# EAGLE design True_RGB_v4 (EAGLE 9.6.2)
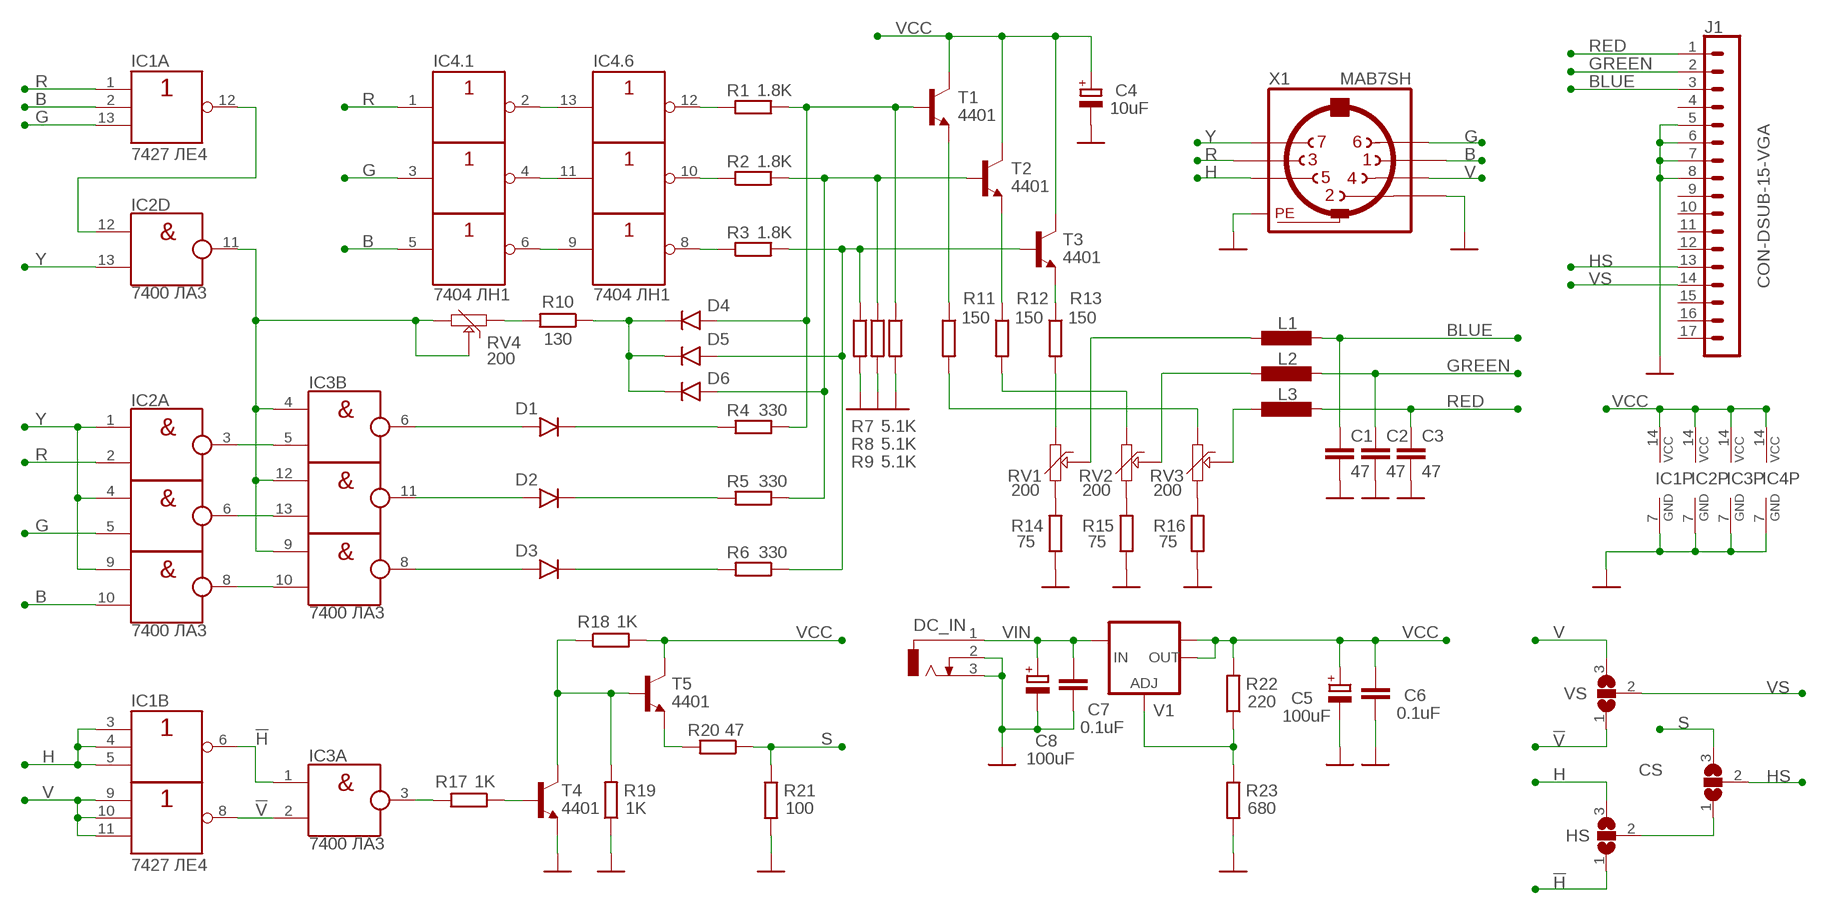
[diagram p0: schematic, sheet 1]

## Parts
C1  47  C-EU050-024X044  [C050-024X044]
C2  47  C-EU050-024X044  [C050-024X044]
C3  47  C-EU050-024X044  [C050-024X044]
C4  10uF  CPOL-EUE2.5-6  [E2,5-6]
C5  100uF  CPOL-EUE2.5-6  [E2,5-6]
C6  0.1uF  C-EU050-024X044  [C050-024X044]
C7  0.1uF  C-EU050-024X044  [C050-024X044]
C8  100uF  CPOL-EUE2.5-6  [E2,5-6]
CS  SJ2W  [SJ_2]
D1  1N4148AS  [D4148-2]
D2  1N4148AS  [D4148-2]
D3  1N4148AS  [D4148-2]
D4  1N4148AS  [D4148-2]
D5  1N4148AS  [D4148-2]
D6  1N4148AS  [D4148-2]
DC_IN  DCJ0202  [DCJ0202]
HS  SJ2W  [SJ_2]
IC1  7427 ЛЕ4  74HC27N  [DIL14]
IC2  7400 ЛА3  74HC00N  [DIL14]
IC3  7400 ЛА3  74HC00N  [DIL14]
IC4  7404 ЛН1  74HC04N  [DIL14]
J1  CON-DSUB-15-VGA  [181-015-212-171]
L1  0.56uH  L-EU0207/12  [0207/12]
L2  0.56uH  L-EU0207/12  [0207/12]
L3  0.56uH  L-EU0207/12  [0207/12]
R1  1.8K  R-EU_0207/2V  [0207/2V]
R2  1.8K  R-EU_0207/2V  [0207/2V]
R3  1.8K  R-EU_0207/2V  [0207/2V]
R4  330  R-EU_0207/2V  [0207/2V]
R5  330  R-EU_0207/2V  [0207/2V]
R6  330  R-EU_0207/2V  [0207/2V]
R7  5.1K  R-EU_0207/2V  [0207/2V]
R8  5.1K  R-EU_0207/2V  [0207/2V]
R9  5.1K  R-EU_0207/2V  [0207/2V]
R10  130  R-EU_0207/2V  [0207/2V]
R11  150  R-EU_0207/2V  [0207/2V]
R12  150  R-EU_0207/2V  [0207/2V]
R13  150  R-EU_0207/2V  [0207/2V]
R14  75  R-EU_0207/2V  [0207/2V]
R15  75  R-EU_0207/2V  [0207/2V]
R16  75  R-EU_0207/2V  [0207/2V]
R17  1K  R-EU_0207/2V  [0207/2V]
R18  1K  R-EU_0207/2V  [0207/2V]
R19  1K  R-EU_0207/2V  [0207/2V]
R20  47  R-EU_0207/2V  [0207/2V]
R21  100  R-EU_0207/2V  [0207/2V]
R22  220  R-EU_0207/2V  [0207/2V]
R23  680  R-EU_0207/2V  [0207/2V]
RV1  200  TRIM-6MM  [6MM]
RV2  200  TRIM-6MM  [6MM]
RV3  200  TRIM-6MM  [6MM]
RV4  200  TRIM-6MM  [6MM]
T1  4401  2N4401-NPN-TO92-EBC  [TO92-EBC]
T2  4401  2N4401-NPN-TO92-EBC  [TO92-EBC]
T3  4401  2N4401-NPN-TO92-EBC  [TO92-EBC]
T4  4401  2N4401-NPN-TO92-EBC  [TO92-EBC]
T5  4401  2N4401-NPN-TO92-EBC  [TO92-EBC]
V1  LM1117IMPX-ADJ  [SOT223]
VS  SJ2W  [SJ_2]
X1  MAB7SH  [MAB7SH]

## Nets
!H: HS.1 IC1.6(B:O) IC3.1(A:I0)
!V: IC1.8(C:O) IC3.2(A:I1) VS.1
B: IC1.2(A:I1) IC2.10(C:I1) IC4.5(.3:I) X1.1
BLUE: C1.1 J1.3 L1.1
G: IC1.13(A:I2) IC2.5(B:I1) IC4.3(.2:I) X1.6
GND: C1.2 C2.2 C3.2 C4.- C5.- C6.2 C7.2 C8.- DC_IN.2 DC_IN.3 IC1.7(P:GND) IC2.7(P:GND) IC3.7(P:GND) IC4.7(P:GND) J1.5 J1.6 J1.7 J1.8 R7.2 R8.2 R9.2 R14.1 R15.1 R16.1 R19.1 R21.2 R23.2 T4.E X1.2 X1.PE X1.PE@(PE)
GREEN: C2.1 J1.2 L2.1
H: HS.3 IC1.3(B:I0) IC1.4(B:I1) IC1.5(B:I2) X1.5
HS: CS.2 J1.13
N$1: D3.C R6.2
N$2: D2.C R5.2
N$3: D1.C R4.2
N$4: L1.2 RV1.S
N$5: IC1.12(A:O) IC2.12(D:I0)
N$6: CS.1 HS.2
N$7: L2.2 RV2.S
N$8: D5.A R3.2 R6.1 R7.1 T3.B
N$9: D6.A R2.2 R5.1 R8.1 T2.B
N$10: D4.A R1.2 R4.1 R9.1 T1.B
N$11: L3.2 RV3.S
N$12: R14.2 RV1.A
N$13: R15.2 RV2.A
N$14: R16.2 RV3.A
N$15: R11.1 T1.E
N$16: R12.2 RV2.E
N$17: R11.2 RV3.E
N$18: R12.1 T2.E
N$19: IC2.3(A:O) IC3.5(B:I1)
N$20: IC2.6(B:O) IC3.13(D:I1)
N$21: IC2.8(C:O) IC3.10(C:I1)
N$22: D1.A IC3.6(B:O)
N$23: D2.A IC3.11(D:O)
N$24: D3.A IC3.8(C:O)
N$25: IC4.2(.1:O) IC4.13(.6:I)
N$26: IC4.4(.2:O) IC4.11(.5:I)
N$27: IC4.6(.3:O) IC4.9(.4:I)
N$28: IC4.12(.6:O) R1.1
N$29: IC4.10(.5:O) R2.1
N$30: IC4.8(.4:O) R3.1
N$31: IC3.3(A:O) R17.2
N$32: R22.1 R23.1 V1.1(ADJ)
N$34: R17.1 T4.B
N$36: D4.C D5.C D6.C R10.1
N$37: R10.2 RV4.E
N$38: IC2.11(D:O) IC3.4(B:I0) IC3.9(C:I0) IC3.12(D:I0) RV4.A RV4.S
N$39: R13.1 T3.E
N$40: R13.2 RV1.E
N$176: R20.2 T5.E
N$177: R18.1 R19.2 T4.C T5.B
R: IC1.1(A:I0) IC2.2(A:I1) IC4.1(.1:I) X1.3
RED: C3.1 J1.1 L3.1
S: CS.3 R20.1 R21.1
V: IC1.9(C:I0) IC1.10(C:I1) IC1.11(C:I2) VS.3 X1.4
VCC: C4.+ C5.+ C6.1 IC1.14(P:VCC) IC2.14(P:VCC) IC3.14(P:VCC) IC4.14(P:VCC) R18.2 R22.2 T1.C T2.C T3.C T5.C V1.2(OUT) V1.TAB(OUT1)
VIN: C7.1 C8.+ DC_IN.1 V1.3(IN)
VS: J1.14 VS.2
Y: IC2.1(A:I0) IC2.4(B:I0) IC2.9(C:I0) IC2.13(D:I1) X1.7
Unconnected: J1.4 J1.9 J1.10 J1.11 J1.12 J1.15 J1.16 J1.17

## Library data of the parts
C1-C3 C6 C7 = rcl:C-EU: CAPACITOR, European symbol; SPICEPREFIX: C
C4 C5 C8 = rcl:CPOL-EU: POLARIZED CAPACITOR, European symbol; SPICEPREFIX: C
CS HS VS = jumper:SJ2W: SMD solder JUMPER
D1-D6 = 27C322:1N4148
DC_IN = power_jack:DCJ0202: DC POWER JACK Source: DCJ0202.pdf; OC_FARNELL: unknown; OC_NEWARK: unknown
IC1 = 74xx-eu:74*27: Triple 3-input NOR gate
IC2 IC3 = 74xx-eu:74*00: Quad 2-input NAND gate
IC4 = 74xx-eu:74*04: Hex INVERTER
J1 = m-pad-2.1:CON-DSUB-15-VGA: NORCOMP's High Density 90° PC Mount D-Sub Connector 181 Series: SPECIFICATIONS: Contact Rating: 5 Amps Dielectric Strength: 1000V AC RMS Insulation Resistance: 1000 meg ohms Contact Material: Phosphor Bronze Contact Finish: Gold flash over Nickel Operating Temperature: -55°C to 150°C Shell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
L1-L3 = rcl:L-EU: INDUCTOR, European symbol; SPICEPREFIX: L
R1-R23 = rcl:R-EU_: RESISTOR, European symbol; SPICEPREFIX: R
RV1-RV4 = 27C322:TRIM-6MM
T1-T5 = transistor-neu-to92:*-NPN-: NPN Transistror
V1 = lm1117:LM1117IMPX-ADJ
X1 = con-hirschmann:MAB7SH: Female CONNECTOR 7 pins with shield, horizontal (DIN 45329); OC_FARNELL: unknown; OC_NEWARK: unknown

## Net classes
1 power: width 0.66 mm, clearance 0.254 mm

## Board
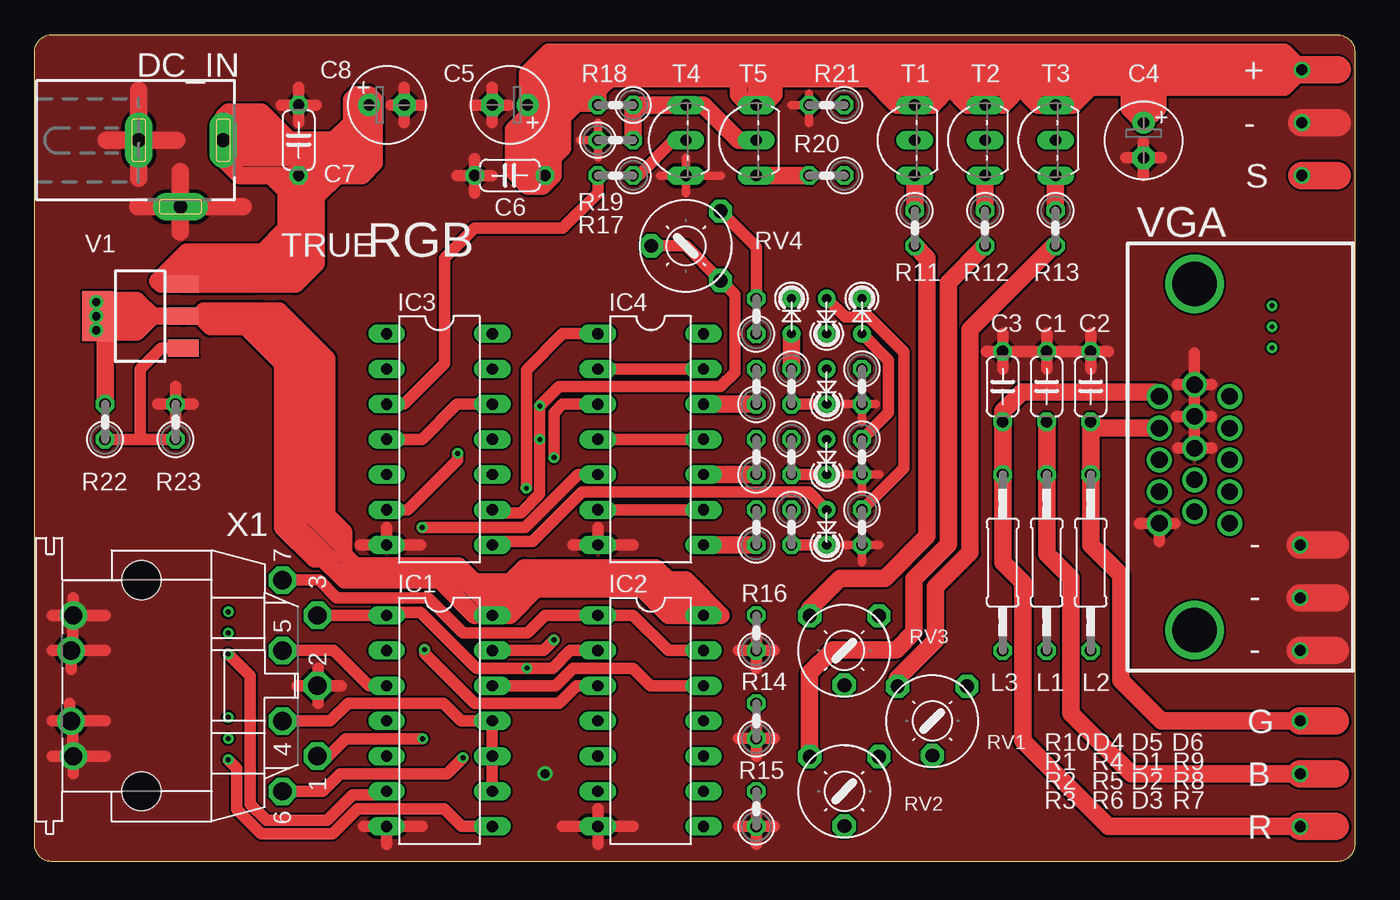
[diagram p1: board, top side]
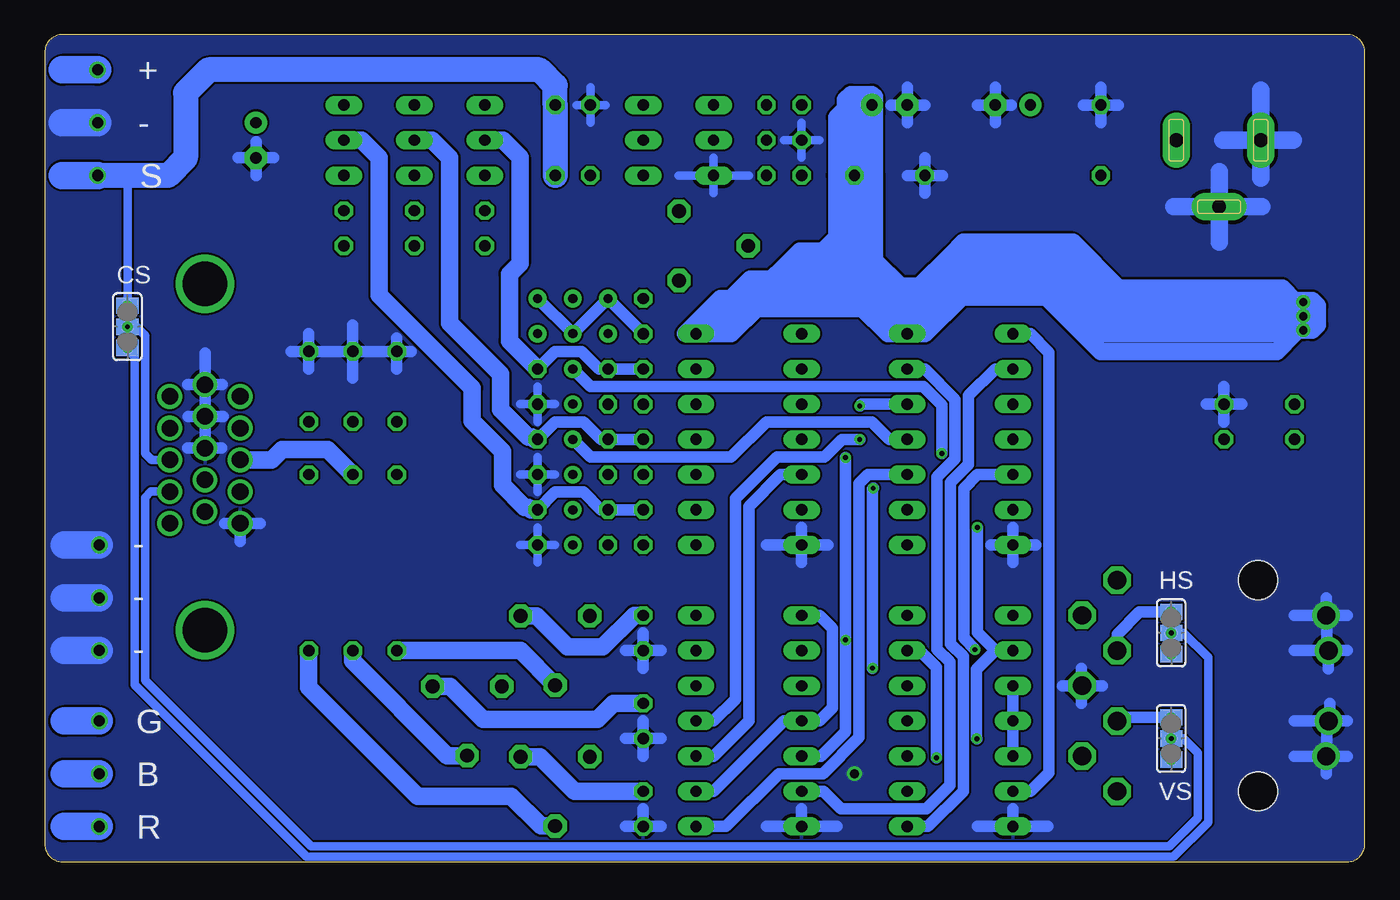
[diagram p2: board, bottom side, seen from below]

Size 95.25 x 59.69 mm. Coordinates in mm from the lower left corner, seen from the top.
Outline: 1.27,59.69 93.98,59.69 arc-90 95.25,58.42 95.25,1.27 arc-90 93.98,0 1.27,0 arc-90 0,1.27 0,58.42 arc-90 1.27,59.69
Copper layers (1*16): Top 0.035mm / dielectric 1.5mm / Bottom 0.035mm
Design rules "default *": minimum track width 6mil, minimum drill 0.35mm, track to track 6mil, track to pad 6mil, pad to pad 6mil, via to via 6mil, smd to smd 6mil, copper to edge 2mil, drill to drill 6mil, minimum pad ring 10mil, minimum via ring 8mil, stop-mask expansion 4mil, vias tented up to drill 20mil, thermal gap 10mil

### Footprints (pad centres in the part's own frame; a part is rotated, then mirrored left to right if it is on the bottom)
C050-024X044 = drill 0.813 octagon: 1 -2.54,0; 2 2.54,0
E2,5-6 = drill 0.813 pad 1.6: + -1.27,0 | drill 0.813 pad 1.6 octagon: - 1.27,0
SJ_2 = smd 1.168 x 1.6: 1 -1.524,0; 2 0,0; 3 1.524,0
D4148-2 = drill 0.65 pad 1.27: A 1.27,0; C -1.27,0
DCJ0202 = drill 1 pad 2 long: 1 0,3.1; 2 4.8,0; 3 0,-3
DIL14 = drill 0.813 long: 1 -7.62,-3.81; 2 -5.08,-3.81; 3 -2.54,-3.81; 4 0,-3.81; 5 2.54,-3.81; 6 5.08,-3.81; 7 7.62,-3.81; 8 7.62,3.81; 9 5.08,3.81; 10 2.54,3.81; 11 0,3.81; 12 -2.54,3.81; 13 -5.08,3.81; 14 -7.62,3.81
181-015-212-171 = drill 1.194: 1 4.371,2.541; 2 2.08,2.541; 3 -0.211,2.541; 4 -2.502,2.541; 5 -4.793,2.541; 6 5.217,0; 7 2.926,0; 8 0.635,0; 9 -1.656,0; 10 -3.947,0; 11 4.371,-2.541; 12 2.08,-2.541; 13 -0.211,-2.541; 14 -2.502,-2.541; 15 -4.793,-2.541 | drill 3.2: 16 -12.502,0; 17 12.502,0
0207/12 = drill 0.813 octagon: 1 -6.35,0; 2 6.35,0
0207/2V = drill 0.813 octagon: 1 -1.27,0; 2 1.27,0
6MM = drill 1 pad 1.676 octagon: A -2.5,-2.5; E 2.5,-2.5; S 0,2.5
TO92-EBC = drill 0.813 long: B 0,-1.27; C 2.54,-1.27; E -2.54,-1.27
SOT223 = smd 1.219 x 2.235: 1 -2.311,-3.099; 2 0,-3.099; 3 2.311,-3.099 | smd 3.6 x 2.2: TAB 0,3.099
MAB7SH = drill 1.321 octagon: 1 5.08,12.7; 2 0,12.7; 3 -5.08,12.7; 4 2.54,10.16; 5 -2.54,10.16; 6 7.62,10.16; 7 -7.62,10.16 | drill 1.321: PE -2.54,-5.08; PE@ 2.54,-5.08 | hole 2.794: 7.62,0; -7.62,0

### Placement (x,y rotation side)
C1  73.03,34.29 90 top
C2  76.2,34.29 90 top
C3  69.85,34.29 90 top
C4  80.01,52.07 270 top
C5  34.29,54.61 180 top
C6  34.29,49.53 180 top
C7  19.05,52.07 90 top
C8  25.4,54.61 0 top
CS  89.28,38.61 90 bottom
D1  57.15,34.29 90 top
D2  57.15,29.21 90 top
D3  57.15,24.13 90 top
D4  54.61,39.37 270 top
D5  57.15,39.37 90 top
D6  59.69,39.37 270 top
DC_IN  10.52,52.07 270 top
HS  13.97,16.51 90 bottom
IC1  29.21,10.16 270 top
IC2  44.45,10.16 270 top
IC3  29.21,30.48 270 top
IC4  44.45,30.48 270 top
J1  83.69,29.21 90 top
L1  73.03,21.59 270 top
L2  76.2,21.59 270 top
L3  69.85,21.59 270 top
R1  52.07,34.29 90 top
R2  52.07,29.21 90 top
R3  52.07,24.13 90 top
R4  54.61,34.29 270 top
R5  54.61,29.21 270 top
R6  54.61,24.13 270 top
R7  59.69,24.13 270 top
R8  59.69,29.21 270 top
R9  59.69,34.29 270 top
R10  52.07,39.37 90 top
R11  63.5,45.72 270 top
R12  68.58,45.72 270 top
R13  73.66,45.72 270 top
R14  52.07,10.16 90 top
R15  52.07,3.81 90 top
R16  52.07,16.51 90 top
R17  41.91,49.53 180 top
R18  41.91,54.61 180 top
R19  41.91,52.07 0 top
R20  57.15,49.53 180 top
R21  57.15,54.61 180 top
R22  5.08,31.75 90 top
R23  10.16,31.75 90 top
RV1  64.77,10.16 180 top
RV2  58.42,5.08 180 top
RV3  58.42,15.24 180 top
RV4  46.99,44.45 90 top
T1  62.23,52.07 90 top
T2  67.31,52.07 90 top
T3  72.39,52.07 90 top
T4  45.72,52.07 90 top
T5  50.8,52.07 90 top
V1  7.62,39.37 90 top
VS  13.97,8.89 90 bottom
X1  7.71,12.7 270 top

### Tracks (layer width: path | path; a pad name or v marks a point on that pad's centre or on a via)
!H  (via drill 0.35)
  Top 0.813: IC1.6 25.15,4.83 22.95,4.83 21.11,2.98 16.73,2.98 15.56,4.16 15.56,13.4 HS.1
  Bottom 0.813: IC3.1 24.13,38.1 22.78,36.75 22.78,6.43 24.13,5.08 IC1.6
  other vias: 13.97,14.99
!V  (via drill 0.35)
  Top 0.813: IC1.8 30.81,2.54 29.54,3.81 23.3,3.81 21.51,2.02 16.33,2.02 14.58,3.77 14.58,6.76 VS.1
  Bottom 0.813: IC1.8 31.52,2.54 28.98,5.08 28.98,14.82 29.9,15.73 29.9,27.37 28.6,28.66 28.6,33.63 26.67,35.56 IC3.2
  other vias: 13.97,7.37
B  (via drill 0.35)
  Top 0.813: IC4.5 39.21,27.94 35.4,24.13 v27.97,24.13 | v28,8.88 22.43,8.88 21.17,7.62 X1.1
  Bottom 0.813: IC2.10 46.99,7.62 44.45,10.16 44.45,25.65 42.16,27.94 IC4.5 | IC1.2 26.64,15.24 | v27.97,24.13 v27.96,24.13 27.96,16.56 26.64,15.24 | 26.64,15.24 28.01,13.87 28.01,8.89 v28,8.88
BLUE  (via drill 0.8)
  Top 1.27: C1.1 L1.1 73.03,22.23 74.75,20.5 74.75,10.72 79.12,6.35 v91.31,6.35
  Top 2: v91.31,6.35 93.85,6.35
  Bottom 1.27: L1.1 74.85,29.76 78.1,29.76 78.87,29 J1.3
  Bottom 2: v91.31,6.35 93.85,6.35
G  (via drill 0.35)
  Top 0.813: IC4.3 38.09,33.02 37.47,32.4 v37.47,29.16 | X1.6 20.78,5.08 22.05,6.35 29.76,6.35 v30.91,7.5 | v37.47,16 36.7,15.24 IC1.13
  Bottom 0.813: IC2.5 39.23,7.62 37.47,9.38 v37.47,16 v37.47,29.16 | v30.91,7.5 30.91,14.02 32.13,15.24 IC1.13
GND  (via drill 0.65, 0.8, 1.3 pad 2)
  Top 0.61: R9.2 60.71,33.02 | R9.2 59.69,34.29 | R9.2 58.42,33.02 | R9.2 59.69,31.75 | R8.2 60.96,27.94 | R8.2 59.69,29.21 | R8.2 58.42,27.94 | R8.2 59.69,26.67 | R7.2 60.96,22.86 | R7.2 59.69,24.13 | R7.2 58.42,22.86 | R7.2 59.69,21.59 | T4.E 46.99,48.26 | T4.E 45.11,49.53 | T4.E 49.53,49.53 | T4.E 46.99,50.8 | R21.2 55.88,53.29 | R21.2 54.61,54.61 | R21.2 57.15,54.61 | R19.1 39.37,52.07 | R19.1 40.64,53.34 | R19.1 40.64,50.8 | R19.1 41.91,52.07 | R21.2 55.88,55.42
  Top 0.813: C5.- 33.02,55.88 | C5.- 31.75,54.61 | C5.- 34.2,54.61 | C5.- 33.02,53.34 | C6.2 31.75,50.75 | C6.2 30.48,49.53 | C6.2 33.02,49.53 | C6.2 31.75,48.26 | IC4.7 38.86,22.86 | IC4.7 40.64,24.13 | IC4.7 43.18,22.86 | C4.- 80.01,51.98 | C4.- 80.01,49.53 | C4.- 81.28,50.8 | C4.- 78.74,50.8 | C3.2 69.85,38.1 | C3.2 C1.2 | C3.2 69.85,35.56 | C1.2 73.03,35.56 | C1.2 73.03,38.1 | C2.2 C1.2 | C2.2 77.47,36.83 | C2.2 76.2,38.1 | C2.2 76.2,35.56 | C3.2 68.68,36.83 | R16.1 50.8,15.24 | R16.1 52.07,16.51 | R16.1 53.34,15.24 | R16.1 52.07,13.97 | R14.1 52.07,7.62 | R14.1 52.07,10.16 | R14.1 50.8,8.89 | R14.1 53.34,8.89 | R15.1 52.07,3.81 | R15.1 52.07,1.27 | R15.1 53.34,2.54 | R15.1 50.8,2.54 | IC2.7 38.1,2.54 | IC2.7 43.18,2.54 | IC2.7 40.64,1.27 | IC2.7 40.64,3.81 | IC1.7 27.94,2.54 | IC1.7 25.4,1.27 | IC3.7 27.84,22.86 | IC3.7 25.4,24.13 | X1.2 18.92,12.7 | 20.45,13.97 20.45,12.74 X1.2 | X1.2 20.45,12.66 20.45,11.43 | X1.2 22.1,12.7 | v2.79,7.62 1.27,7.62 | v2.79,7.62 5.08,7.62 | X1.PE@ 5.08,10.16 | X1.PE@ 1.27,10.16 | X1.PE@ 2.54,10.25 2.54,11.43 | X1.PE@ 2.76,10.03 2.76,7.66 v2.79,7.62 | v2.79,7.62 2.79,6.35 | X1.PE 2.63,13.88 | X1.PE 2.76,15.37 2.76,17.74 v2.79,17.78 | X1.PE 1.27,15.24 | X1.PE 5.08,15.24 | v2.79,17.78 5.08,17.78 | v2.79,17.78 1.27,17.78 | v2.79,17.78 2.79,19.05 | R23.2 10.16,34.29 | R23.2 10.16,31.75 | R23.2 11.43,33.02 | R23.2 8.89,33.02 | C7.2 19.05,55.88 | C7.2 19.05,53.34 | C7.2 20.32,54.61 | C7.2 17.78,54.61 | C8.- 26.67,55.88 | C8.- 27.94,54.61 | C8.- 26.67,53.34 | C8.- 25.7,54.61 | J1.6 J1.7 | J1.7 J1.8 | J1.6 83.69,36.7 | J1.6 84.95,34.43 | J1.6 82.43,34.43 | J1.8 82.49,29.84 | J1.8 84.92,29.84 | J1.7 82.36,32.14 | J1.7 84.9,32.14 | J1.5 81.15,23.11 | J1.5 79.72,24.42 | J1.5 82.26,24.42 | IC1.7 23.75,2.54 | IC3.7 23.5,22.86
  Top 1.27: DC_IN.3 7.52,55.67 | DC_IN.3 7.52,49.32 | DC_IN.3 10.26,52.07 | DC_IN.3 5.18,52.07 | DC_IN.2 10.52,49.78 | DC_IN.2 10.52,45.45 | DC_IN.2 7.44,47.27 | DC_IN.2 15.06,47.27
  Top 2: v91.44,53.34 93.98,53.34 | v91.31,15.24 93.85,15.24 | v91.31,19.05 93.85,19.05 | v91.31,22.86 93.85,22.86
  Bottom 0.61: R19.1 40.64,53.34 | R19.1 39.37,52.07 | R19.1 41.91,52.07 | R19.1 40.64,50.8 | T4.E 44.45,49.53 | T4.E 46.99,50.8 | T4.E 46.99,48.26 | T4.E 49.53,49.53 | R21.2 56.9,54.61 | R21.2 55.88,53.34 | R21.2 54.8,54.61 | R21.2 55.88,55.88 | R8.2 59.69,29.21 | R8.2 58.42,27.94 | R8.2 60.96,27.94 | R8.2 59.69,26.67 | R7.2 59.69,21.59 | R7.2 60.96,22.86 | R7.2 58.42,22.86 | R7.2 59.69,24.13 | R9.2 59.69,34.29 | R9.2 60.96,33.02 | R9.2 58.42,33.02 | R9.2 59.69,31.75
  Bottom 0.813: C6.2 30.48,49.53 | C6.2 33.02,49.53 | C6.2 31.75,50.8 | C5.- 33.02,55.88 | C5.- 34.2,54.61 | C5.- 31.75,54.61 | C5.- 33.02,53.34 | C4.- 78.74,50.8 | C4.- 80.01,49.53 | C4.- 81.28,50.8 | C4.- 80.01,51.98 | C3.2 68.83,36.83 | C3.2 C1.2 | C1.2 C2.2 | C2.2 77.47,36.83 | C2.2 76.2,38.1 | C2.2 76.2,35.56 | C1.2 73.03,38.73 | C1.2 73.03,34.92 | C3.2 69.85,37.8 | C3.2 69.85,35.56 | R16.1 52.07,13.97 | R16.1 50.8,15.24 | R16.1 53.34,15.24 | R16.1 52.07,16.51 | R14.1 52.07,10.16 | R14.1 53.34,8.89 | R14.1 50.8,8.89 | R14.1 52.07,7.62 | R15.1 50.8,2.54 | R15.1 52.07,3.81 | R15.1 53.34,2.54 | v2.79,7.62 5.08,7.62 | v2.79,7.62 1.27,7.62 | v2.79,7.62 2.79,6.35 | v2.79,7.62 2.76,7.66 2.76,10.03 X1.PE@ | X1.PE@ 2.54,10.25 2.54,11.43 | X1.PE 2.63,13.93 | X1.PE 2.76,15.37 2.76,17.74 v2.79,17.78 | v2.79,17.78 5.08,17.78 | v2.79,17.78 1.27,17.78 | v2.79,17.78 2.79,19.05 | X1.PE 5.08,15.24 | X1.PE 1.27,15.24 | X1.PE@ 5.08,10.16 | X1.PE@ 1.27,10.16 | X1.2 18.92,12.7 | 20.45,13.97 20.45,12.74 X1.2 | X1.2 20.45,12.66 20.45,11.43 | X1.2 21.82,12.7 | R23.2 11.43,33.02 | R23.2 8.89,33.02 | R23.2 10.16,34.29 | R23.2 10.16,31.75 | C7.2 19.05,55.88 | C7.2 19.05,53.34 | C7.2 20.32,54.61 | C7.2 17.78,54.61 | C8.- 26.67,55.88 | C8.- 26.67,53.34 | C8.- 25.49,54.61 | C8.- 27.94,54.61 | C6.2 31.75,48.26 | IC2.7 43.18,2.54 | IC2.7 40.64,3.81 | IC2.7 38.1,2.54 | IC1.7 27.94,2.54 | IC1.7 25.4,3.81 | IC1.7 22.86,2.54 | IC3.7 25.4,21.59 | IC3.7 25.4,24.13 | IC3.7 27,22.86 | IC3.7 23.75,22.86 | IC4.7 38.73,22.86 | IC4.7 40.64,24.13 | IC4.7 43.18,22.86 | IC4.7 40.64,21.59 | J1.6 J1.7 | J1.7 J1.8 | J1.6 83.69,36.7 | J1.6 84.95,34.43 | J1.6 82.43,34.43 | J1.8 82.49,29.84 | J1.8 84.92,29.84 | J1.7 82.36,32.14 | J1.7 84.9,32.14 | J1.5 81.15,23.11 | J1.5 79.72,24.42 | J1.5 82.26,24.42
  Bottom 1.27: DC_IN.3 7.52,55.67 | DC_IN.3 7.52,49.32 | DC_IN.2 10.52,49.78 | DC_IN.2 10.52,44.7 | DC_IN.2 13.79,47.27 | DC_IN.2 7.44,47.27 | DC_IN.3 5.18,52.07 | DC_IN.3 10.26,52.07
  Bottom 2: v91.44,53.34 93.98,53.34 | v91.31,15.24 93.85,15.24 | v91.31,19.05 93.85,19.05 | v91.31,22.86 93.85,22.86
  other vias: 36.83,6.35
  pour Bottom: -2.54,62.23 97.79,62.23 97.79,-2.54 -2.54,-2.54
  pour Top: -2.54,62.23 97.79,62.23 97.79,-2.54 -2.54,-2.54
GREEN  (via drill 0.8)
  Top 1.27: J1.2 76.71,31.29 76.2,31.8 C2.1 L2.1 76.2,22.86 78.36,20.7 78.36,13.08 81.28,10.16 v91.31,10.16
  Top 2: v91.31,10.16 93.85,10.16
  Bottom 2: v91.31,10.16 93.85,10.16
H  (via drill 0.35)
  Top 0.813: IC1.3 24.13,12.7 21.59,15.24 X1.5
  Bottom 0.813: IC1.3 IC1.4 IC1.5 | HS.3 16.26,18.03 17.87,16.42 X1.5
  other vias: 13.97,18.03
HS  (via drill 0.35)
  Bottom 0.61: J1.13 87.55,29 88.01,29.46 88.01,37.97 88.65,38.61 CS.2
  other vias: 89.28,38.61
N$1
  Top 0.813: R6.2 D3.C
N$2
  Top 0.813: R5.2 D2.C
N$3
  Top 0.813: R4.2 D1.C
N$4
  Bottom 1.27: L1.2 73.03,14.48 66.21,7.66 RV1.S
N$5
  Top 0.813: IC2.12 44.45,12.7 43.18,13.97 38.86,13.97 37.59,12.7 IC1.12
N$6  (via drill 0.35)
  Bottom 0.61: HS.2 13.08,16.51 11.3,14.73 11.3,2.86 13.81,0.36 76.36,0.36 88.77,12.77 88.77,36.45 89.28,36.96 CS.1
  other vias: 13.97,16.51 89.28,37.08
N$7
  Bottom 1.27: L2.2 76.2,12.57 68.37,4.74 61.59,4.74 59.44,2.58 RV2.S
N$8
  Top 0.813: D5.A 58.5,39.29 60.18,39.29 62.71,36.77 62.71,28.42 R7.1
  Bottom 0.813: R3.2 R6.1 55.12,25.4 56.39,26.67 58.42,26.67 R7.1
  Bottom 1.27: R7.1 60.18,25.4 60.35,25.58 60.63,25.58 62.23,27.18 62.23,29.61 64.41,31.8 64.41,34.19 71.12,40.89 71.12,50.8 72.39,52.07 T3.B
N$9
  Top 0.813: D6.A 61.62,36.17 61.62,32.41 R8.1
  Bottom 0.813: R2.2 R5.1 55.12,30.48 56.39,31.75 58.42,31.75 R8.1
  Bottom 1.27: R8.1 59.92,30.48 60.1,30.66 60.38,30.66 62.36,32.64 62.36,35.18 66.04,38.86 66.04,50.8 67.31,52.07 T2.B
N$10
  Top 1.27: D4.A R4.1
  Bottom 0.813: R1.2 R4.1 55.24,35.56 56.52,36.83 58.42,36.83 R9.1
  Bottom 1.27: R9.1 61.72,37.59 61.72,42.42 60.96,43.18 60.96,50.84 62.19,52.07 T1.B
N$11
  Bottom 1.27: RV3.S 60.92,15.24 L3.2
N$12
  Bottom 1.27: R14.2 54.23,11.43 55.37,10.29 63.63,10.29 66,12.66 RV1.A
N$13
  Bottom 1.27: RV2.A 59.52,7.58 57.02,5.08 R15.2
N$14
  Bottom 1.27: RV3.A 59.78,17.74 57.53,15.49 54.99,15.49 52.7,17.78 R16.2
N$15
  Top 1.27: T1.E R11.1
N$16
  Top 1.27: R12.2 65.94,41.81 65.94,22.91 63.44,20.4 63.44,16.57 62.17,15.3 57.59,15.3 55.92,13.63 RV2.E
N$17
  Top 1.27: R11.2 64.39,43.56 64.39,23.5 61.34,20.45 58.12,20.45 55.92,18.25 RV3.E
N$18
  Top 1.27: R12.1 T2.E
N$19  (via drill 0.35)
  Top 0.813: IC2.3 39.12,12.7 37.85,11.43 31.75,11.43 28.13,15.05 v28.13,15.31
  Bottom 0.813: IC3.5 27.94,27.94 28.93,26.95 28.93,16.14 28.13,15.33 v28.13,15.31
N$20
  Bottom 0.813: IC2.6 39.08,5.08 37.81,3.81 31.64,3.81 29.94,5.5 29.94,14.42 30.86,15.34 30.86,27.77 29.56,29.06 29.56,33.37 31.75,35.56 IC3.13
N$21
  Bottom 0.813: IC2.8 46.1,2.54 42.29,6.35 39.12,6.35 36.5,8.97 36.5,27.3 35.85,27.94 IC3.10
N$22  (via drill 0.35)
  Top 0.813: IC3.6 26.92,25.4 30.53,29 v30.53,29.46
  Bottom 0.813: D1.A 55.88,34.29 31.84,34.29 30.53,32.97 v30.53,29.46
N$23
  Bottom 0.813: D2.A 55.88,29.21 45.72,29.21 43.18,31.75 35.56,31.75 34.29,30.48 IC3.11
N$24
  Top 0.813: D3.A 55.88,26.67 39.5,26.67 35.93,23.1 33.26,23.1 IC3.8
N$25
  Top 0.813: IC4.2 IC4.13
N$26
  Top 0.813: IC4.4 IC4.11
N$27
  Top 0.813: IC4.6 IC4.9
N$28
  Top 1.27: IC4.12 R1.1
N$29
  Top 1.27: IC4.10 R2.1
N$30
  Top 1.27: IC4.8 R3.1
N$31
  Top 0.813: IC3.3 26.67,33.02 29.59,35.94 29.59,43.56 31.75,45.72 38.1,45.72 40.64,48.26 R17.2
N$32
  Top 0.813: V1.1 10.71,37.07 9.13,37.07 7.62,35.56 7.62,30.48 | R23.1 7.62,30.48 | 7.62,30.48 R22.1
N$34
  Top 0.813: R17.1 43.56,49.53 46.1,52.07 T4.B
N$36
  Bottom 0.813: R10.1 D4.C D5.C D6.C
N$37
  Top 0.813: R10.2 52.07,44.37 RV4.E
N$38  (via drill 0.35)
  Top 0.813: IC3.9 33.24,25.18 35.09,25.18 36.45,26.54 v36.45,30.48 v36.45,32.89 37.85,34.29 49.5,34.29 50.52,35.31 50.52,40.92 RV4.A 46.99,44.45 RV4.S | IC3.12 30.48,33.02 27.94,30.48 IC3.4
  Bottom 0.813: IC2.11 46.99,10.16 45.43,11.72 45.43,26.2 42.42,29.21 38.99,29.21 37.72,30.48 v36.45,30.48 | IC3.12 36.32,33.02 v36.45,32.89
N$39
  Top 1.27: T3.E R13.1
N$40
  Top 1.27: R13.2 73.53,44.45 67.49,38.41 67.49,22.32 64.99,19.82 64.99,15.96 62.27,13.25 RV1.E
  Bottom 1.27: R13.2 73.7,44.41
N$176
  Top 1.27: R20.2 T5.E
N$177
  Top 1.27: T5.B 50.8,52.07 48.26,54.61 T4.C R18.1 R19.2
R  (via drill 0.35)
  Top 0.813: IC2.2 38.64,15.24 37.37,13.97 v35.52,13.97 31.9,13.97 27.86,18.01 25.63,18.01 IC1.1 X1.3 | IC4.1 38.1,38.1 35.48,35.48 35.48,26.97 v35.47,26.96
  Bottom 0.813: v35.47,26.96 35.53,26.9 35.53,13.98 v35.52,13.97
RED  (via drill 0.8)
  Top 1.27: J1.1 80.82,33.91 71.25,33.91 69.85,32.51 C3.1 L3.1 69.85,21.59 71.3,20.14 71.3,8.71 77.47,2.54 v91.31,2.54
  Top 2: v91.31,2.54 93.85,2.54
  Bottom 2: v91.31,2.54 93.85,2.54
S  (via drill 0.35, 0.8)
  Top 2: 93.98,49.53 v91.44,49.53
  Bottom 0.61: v91.44,49.53 89.28,49.53 CS.3
  Bottom 1.8: v91.44,49.53 86.36,49.53 85.09,50.8 85.09,55.5 83.44,57.15 59.56,57.15 58.42,56.01 R21.1 R20.1
  Bottom 2: v91.44,49.53 93.98,49.53
  other vias: 89.28,40.13
V  (via drill 0.35)
  Top 0.813: IC1.9 IC1.10 IC1.11 30.77,10.16 29.5,11.43 22.61,11.43 21.34,10.16 X1.4
  Bottom 0.813: VS.3 17.61,10.41 X1.4
  other vias: 13.97,10.41
VCC  (via drill 0.6 pad 0.95, 0.8)
  Top 0.61: V1.TAB v4.44,39.37
  Top 0.813: 5.08,38.11 4.84,38.35 v4.44,38.35
  Top 1.27: 40.64,57.15 78.99,57.15 | 78.99,57.15 81.03,57.15 | 81.03,57.15 82.55,57.15 | 40.64,57.15 40.64,57.4 37.08,57.4 36.2,56.52 | 40.64,57.15 40.64,55.88 | 40.64,55.88 40.88,55.88 41.51,56.52 50.8,56.52 | 50.8,56.52 52.07,56.52 | 52.07,56.52 53.34,56.52 | 53.34,56.52 60.33,56.52 | 60.33,56.52 60.96,56.52 61.59,55.88 66.04,55.88 | T5.C 52.07,56.52 | T5.C 52.58,54.61 53.34,55.37 53.34,56.52 | T5.C 51.56,54.61 50.8,55.37 50.8,56.52 | 35.56,53.85 C5.+ 35.56,55.88 | 36.7,54.61 36.7,56.13 | 35.56,55.88 35.56,56.9 37.07,58.41 82.55,58.41 | 36.2,56.52 35.56,55.88 | 36.7,54.61 36.45,54.36 36.45,49.91 C6.1 | 36.7,54.61 37.4,55.31 | 40.64,55.88 37.4,55.88 37.4,55.31 | 36.2,56.52 38.1,56.52 | 38.1,56.52 40.01,56.52 40.64,57.15 | 35.56,53.85 34.54,52.83 34.54,49.78 35.56,48.77 36.64,48.77 37.4,49.53 | C6.1 36.7,49.66 | C6.1 37.4,49.53 | 37.4,49.53 37.4,50.8 | 37.4,50.8 37.4,55.31 | C6.1 35.56,49.53 35.56,53.85 | T2.C 67.31,54.61 66.04,55.88 | 71.12,55.88 69.85,54.61 | 71.12,55.88 72.39,54.61 T3.C 74.93,54.61 76.2,55.88 | 82.55,55.88 82.55,57.15 | 82.55,57.15 82.55,58.41 | 66.04,55.88 64.77,54.61 T1.C 62.23,54.61 60.33,56.52 | 66.04,55.88 71.12,55.88 | 71.12,55.88 76.2,55.88 | 82.55,58.41 90.18,58.41 v91.44,57.15 90.17,55.88 82.55,55.88 | 82.55,55.88 83.82,57.15 | 76.2,55.88 80.01,55.88 | 80.01,55.88 82.55,55.88 | 40.64,55.88 R18.2 40.51,54.74 39.12,54.74 38.1,53.72 | 38.1,56.52 38.1,53.72 | 38.1,53.72 38.1,51.5 37.4,50.8 | C4.+ 80.01,55.88 | C4.+ 78.99,54.36 78.99,57.15 | C4.+ 81.03,54.36 81.03,57.15 | 8.51,39.37 V1.2 11.94,39.37 | 8.51,39.37 V1.TAB | V1.TAB 5.66,40.51 7.37,40.51 8.51,39.37 | V1.TAB 4.52,38.66 4.95,38.23 7.37,38.23 8.51,39.37
  Top 1.27: 45.72,20.32 44.83,21.21 36.45,21.21 | 36.45,21.21 35.56,20.32 | 35.56,20.32 34.16,18.92 32.38,18.92 29.97,21.34 | 31.75,17.78 29.21,20.32 22.35,20.32 20.83,21.84 | 15.24,38.61 16,38.61 19.05,35.56 19.05,24.13 21.34,21.84 20.83,21.84 | 15.24,38.61 12.7,38.61 11.94,39.37 | 11.94,39.37 12.57,39.37 12.19,39.75 16.38,39.75 | 29.97,21.34 23.11,21.34 22.29,22.16 22.29,22.67 | 22.29,22.67 20.19,24.77 20.19,35.94 16.38,39.75 | 16.38,39.75 17.65,39.75 21.08,36.32 21.08,25.02 22.29,23.81 22.29,22.67 | 15.24,38.61 17.91,35.94 17.91,24.13 20.19,21.84 20.83,21.84 | 35.56,20.32 36.83,20.32 | 36.83,20.32 43.18,20.32 | 43.18,20.32 44.45,20.32 | 44.45,20.32 45.72,20.32 | 45.72,20.32 46.99,20.32 49.53,17.78 IC2.14 | 29.97,21.34 30.61,21.34 31.75,20.19 34.29,20.19 35.31,21.21 36.45,21.21 | R22.2 5.08,38.11 | IC1.14 34.29,17.78 36.2,19.68 | 36.2,19.68 36.83,20.32 | IC2.14 45.72,20.32 | IC2.14 46.99,17.78 44.45,20.32 | IC2.14 45.72,17.78 43.81,19.68 | 43.81,19.68 43.18,20.32 | 36.2,19.68 43.81,19.68
  Top 2: 82.55,57.15 83.82,57.15 v91.44,57.15 93.98,57.15
  Bottom 1.27: v4.44,39.37 19.05,39.37 21.46,41.78 | 21.46,41.78 22.48,42.8 29.59,42.8 32,40.39 34.04,40.39 36.32,42.67 36.32,49.02 C6.1 | v4.44,40.39 4.44,40.51 | 4.44,40.51 5.08,40.51 | 5.08,40.51 18.54,40.51 21.84,43.81 29.84,43.81 | 5.08,38.1 4.83,38.35 v4.44,38.35 3.81,38.35 3.43,38.73 3.43,40.13 3.81,40.51 4.44,40.51 | 5.08,38.1 19.3,38.1 21.97,40.77 22.99,40.77 | 22.99,40.77 29.08,40.77 31.75,38.1 IC3.14 34.42,38.1 36.25,39.93 | 47.75,39.37 45.72,39.37 44.45,40.64 | 44.45,40.64 43.31,41.78 38.1,41.78 | 38.1,41.78 36.7,41.78 34.16,39.24 31.88,39.24 29.34,41.78 21.46,41.78 | 47.75,39.37 49.02,38.1 IC4.14 45.72,38.1 43.89,39.93 36.25,39.93 | 47.75,39.37 46.48,40.64 45.72,40.64 44.32,42.04 42.8,42.04 41.91,42.93 | 36.58,42.93 41.91,42.93 | 41.91,42.93 40.77,44.07 39.12,44.07 | 29.84,43.81 32.13,41.53 33.53,41.53 35.37,43.37 | 35.37,43.37 36.07,44.07 37.47,44.07 | 37.47,44.07 38.1,44.07 | 38.1,44.07 39.12,44.07 | C6.1 35.37,49.53 | 35.37,49.53 35.37,43.37 | C6.1 37.08,49.53 | 37.08,49.53 37.47,49.53 | 37.47,49.53 38.1,49.53 | 37.47,44.07 37.47,45.72 | 37.47,45.72 37.47,49.53 | 38.1,49.53 38.1,44.07 | 37.47,45.72 39.12,44.07 | 5.08,38.1 6.35,36.83 19.05,36.83 22.99,40.77 | 5.08,40.51 5.97,41.4 17.78,41.4 21.08,44.7 28.96,44.7 29.84,43.81 | 35.37,49.53 35.37,54.09 35.4,54.12 35.4,54.61 | 35.4,54.61 C5.+ | C6.1 36.45,49.91 36.45,54.61 C5.+ | 37.08,49.53 37.08,54.61 C5.+ | 37.47,54.36 37.47,54.99 37.08,55.37 35.56,55.37 35.4,55.21 35.4,54.61 | 37.47,54.36 37.47,49.53 | 37.47,54.36 38.1,53.72 38.1,49.53 | 36.25,39.93 36.96,40.64 | 36.96,40.64 38.1,41.78 | 36.96,40.64 44.45,40.64
  Bottom 2: v91.44,57.15 93.98,57.15
VIN
  Top 1.27: 13.62,50.7 14.78,49.53 17.02,49.53 | 13.62,50.7 13.51,50.8 19.05,50.8 | 17.02,49.53 C7.1 | 13.62,50.7 DC_IN.1 18.42,52.07 | C7.1 19.05,50.8 | 19.05,50.8 19.05,52.07 | 18.42,52.07 19.05,52.07 | 13.64,53.77 13.97,54.1 16.38,54.1 17.46,53.02 | 18.42,52.07 17.46,53.02 | 13.64,52.32 14.34,53.02 17.46,53.02 | 19.05,52.07 21.59,52.07 22.86,53.34 22.86,53.98 | 24.13,55.37 23.24,55.37 22.86,54.99 22.86,53.98 | 24.13,55.37 C8.+ 24.13,53.98 | 24.13,55.37 24.51,54.99 24.51,53.98 | 24.51,53.98 24.13,53.98 | 24.13,53.98 22.86,53.98 | 24.51,53.98 24.51,50.42 23.62,49.53 21.84,49.53 | 21.84,49.53 20.07,49.53 | 24.13,52.96 24.13,51.31 23.37,50.55 19.3,50.55 19.05,50.8 | 19.05,50.8 19.94,51.69 22.86,51.69 24.13,52.96 | 24.13,52.96 24.13,53.98 | V1.3 15.77,41.68 | V1.3 9.12,41.68 8.89,41.91 10.99,44.01 16.45,44.01 | 17.02,49.53 18.16,48.39 18.16,45.72 16.45,44.01 | 15.37,42.67 10.39,42.67 11.21,43.5 15.94,43.5 | 15.37,42.67 16.19,43.5 | 15.94,43.5 16.45,44.01 | 20.32,48.01 20.32,43.18 18.82,41.68 V1.3 | 21.84,49.53 20.32,48.01 | 15.37,42.67 15.75,42.29 17.91,42.29 19.05,43.43 19.05,44.96 | C7.1 19.05,44.96 | 15.94,43.5 17.59,43.5 19.05,44.96 | C7.1 20.32,48.26 20.32,48.01
VS  (via drill 0.35)
  Bottom 0.61: J1.14 87.59,26.71 88.01,26.29 88.01,13.08 76.05,1.12 14.12,1.12 12.06,3.18 12.06,7.87 13.08,8.89 VS.2
  other vias: 13.97,8.89
Y
  Top 0.813: IC2.13 45.72,15.24 43.18,17.78 IC2.1 36.83,17.78 35.56,16.51 30.91,16.51 28.37,19.05 21.81,19.05 20.54,20.32 X1.7
  Bottom 0.813: IC2.1 39.37,17.78 38.43,16.84 38.43,11.1 39.37,10.16 IC2.4 41.91,10.16 46.99,5.08 IC2.9

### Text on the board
tPlace: + | - | S | VGA | TRUE | RGB | - | - | - | G | B | R
bPlace: + | - | S | - | - | - | G | B | R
